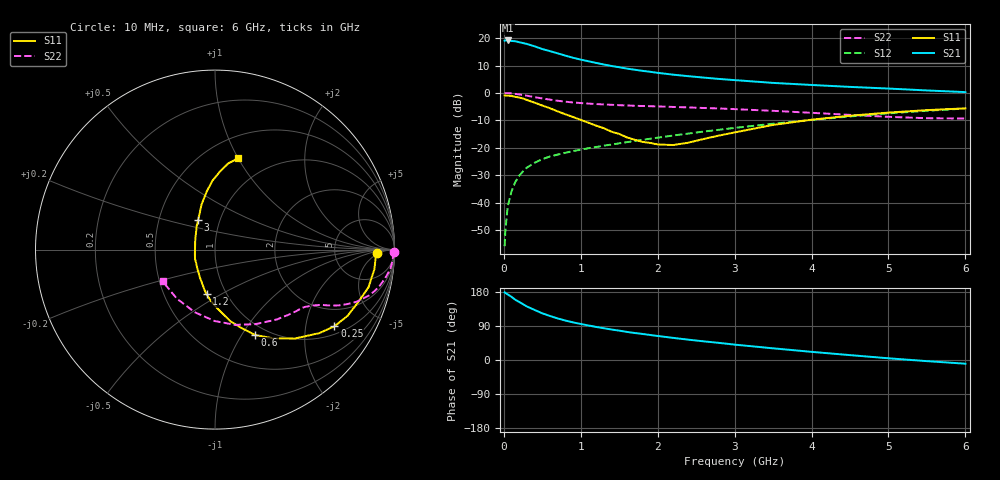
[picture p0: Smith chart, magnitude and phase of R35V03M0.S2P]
! SIEMENS Small Signal Semiconductors
! BFR181
! Si NPN RF Bipolar Junction Transistor in SOT23
! VCE = 5 V  IC = 3 mA
! Common Emitter S-Parameters:  May  1996
# GHz  S  MA  R  50
!  f  S11  S21  S12  S22
! GHz  MAG  ANG  MAG  ANG  MAG  ANG  MAG  ANG
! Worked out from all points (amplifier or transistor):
!   36 points, 10 MHz to 6 GHz, reference 50 ohm
!   highest |S21| = 19.2 dB at 50 MHz (marker M1)
!   |S21| within 3 dB of that: start of sweep to 486.5 MHz
!   unconditionally stable (mu >= 1): 1.39 GHz to 3.215 GHz
!   at 250 MHz: K = 0.30, MSG = 23.4 dB, |S12| = -28.6 dB
!   at 1.4 GHz: K = 1.00, MAG = 14.0 dB, |S12| = -18.8 dB
!   at 6 GHz: K = 0.86, MSG = 3.0 dB, |S12| = -5.7 dB
!   lowest NFmin = 1.40 dB at 450 MHz
!   S11 on the Smith chart (normalised r, x): 10 MHz: 18, -4; 250 MHz: 1.27, -2.90; 600 MHz: 0.87, -1.15; 1.2 GHz: 0.81, -0.43; 3 GHz: 0.79, +0.27; 6 GHz: 0.71, +1.00
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0.01  0.9001 -1.3  9.016 178.5  0.0016 87.5  0.9953 -0.7
0.02  0.8966 -2.4  9.079 176.9  0.0031 85.8  0.9928 -1.3
0.05  0.8947 -7.0  9.086 173.1  0.0084 86.2  0.9919 -3.3
0.1  0.8807 -13.8  8.893 166.6  0.0161 83.0  0.9826 -6.4
0.15  0.8495 -20.2  8.795 158.9  0.0239 77.3  0.9611 -9.6
0.25  0.7906 -32.7  8.133 147.2  0.0373 71.7  0.9184 -14.6
0.3  0.7445 -38.7  7.841 141.2  0.0435 69.7  0.8923 -16.8
0.4  0.6658 -48.1  7.099 132.1  0.0533 65.3  0.8396 -20.3
0.5  0.5905 -56.8  6.334 123.2  0.0619 62.7  0.7948 -22.5
0.6  0.5261 -64.8  5.796 116.1  0.0694 60.6  0.7557 -24.3
0.7  0.4615 -71.3  5.284 109.7  0.075 59.4  0.7208 -25.6
0.8  0.4081 -77.9  4.803 104.1  0.0811 58.5  0.6932 -26.6
0.9  0.3639 -82.6  4.387 99.3  0.0869 58.5  0.6712 -27.3
1.1  0.2864 -94.7  3.788 91.1  0.0981 58.2  0.6401 -29.0
1.2  0.2531 -100.7  3.535 87.3  0.1032 58.5  0.6278 -29.7
1.6  0.1547 -127.0  2.787 74.1  0.1266 59.3  0.5919 -32.8
2.2  0.1121 172.3  2.158 58.4  0.1672 59.4  0.5559 -39.4
3  0.1906 119.3  1.717 40.6  0.2304 56.8  0.5069 -51.3
3.5  0.2611 106.8  1.527 30.8  0.2746 53.7  0.4721 -61.6
4.5  0.3842 92.1  1.291 12.9  0.3731 44.5  0.3981 -90.3
5.5  0.4863 81.2  1.112 -3.0  0.4738 32.2  0.3461 -128.0
6  0.524 75.9  1.037 -9.8  0.5203 25.1  0.3414 -148.9
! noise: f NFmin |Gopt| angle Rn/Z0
0.45  1.4  0.56  17  0.36
0.9  1.5  0.45  35  0.34
1.8  1.85  0.25  82  0.36
